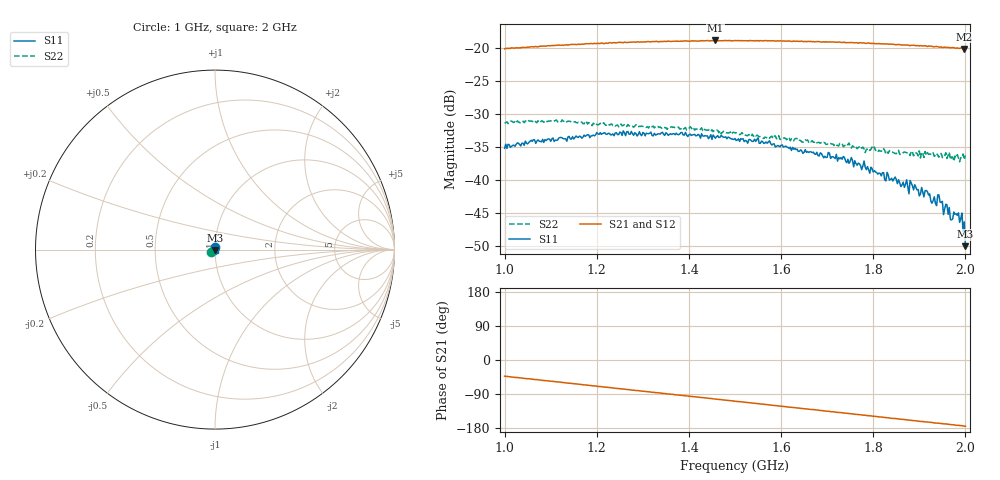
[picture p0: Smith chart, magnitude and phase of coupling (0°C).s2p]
!Agilent Technologies,E8363C,MY43030407,A.09.42.15
!Agilent E8363C: A.09.42.15
!Date: Friday, September 05, 2025 17:32:45
!Correction: S11(Full 2 Port(1,2))
!S21(Full 2 Port(1,2))
!S12(Full 2 Port(1,2))
!S22(Full 2 Port(1,2))
!S2P File: Measurements: S11, S21, S12, S22:
# Hz S  dB  R 50
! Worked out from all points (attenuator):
!   401 points, 1 GHz to 2 GHz, reference 50 ohm
!   highest |S21| = -18.78 dB at 1.458 GHz (marker M1); lowest = -20.1 dB at 1.998 GHz (marker M2)
!   lowest |S11| = -50.1 dB at 2 GHz (marker M3), VSWR 1.01, Z = 49.9 - j0.296 ohm
!   |S11| at or under -10 dB: start of sweep to end of sweep
!   |S22| runs from -37.2 to -30.9 dB; largest |S21 - S12| = 0.0015
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1e9  -35.19 98.9  -20.06 -42.7  -20.03 -42.7  -31.37 -145.9
1.06e9  -34.14 88.2  -19.73 -50.6  -19.74 -50.6  -31.07 -149.8
1.1675e9  -33.66 71.3  -19.34 -64.7  -19.37 -64.9  -31.22 -151.0
1.335e9  -32.98 41.4  -18.99 -86.9  -18.95 -86.9  -32.02 -157.6
1.4575e9  -33.66 18.7  -18.78 -103.1  -18.84 -103.1  -32.53 -157.1
1.5e9  -33.70 12.1  -18.80 -108.8  -18.81 -108.5  -32.85 -157.2
1.545e9  -34.14 -0.2  -18.81 -114.5  -18.83 -114.4  -33.33 -158.1
1.6675e9  -35.86 -26.9  -18.98 -130.8  -18.94 -130.9  -34.03 -157.4
1.75e9  -37.17 -46.5  -19.11 -141.6  -19.12 -141.7  -34.89 -153.4
1.835e9  -40.03 -61.0  -19.36 -152.8  -19.38 -152.9  -35.57 -149.1
1.8725e9  -39.99 -76.6  -19.49 -157.7  -19.48 -158.2  -35.85 -147.9
1.885e9  -40.90 -77.3  -19.51 -159.7  -19.53 -159.1  -35.67 -145.9
1.905e9  -41.15 -84.5  -19.61 -162.4  -19.57 -162.2  -35.81 -144.6
1.9175e9  -41.76 -85.0  -19.72 -163.8  -19.67 -163.5  -35.83 -143.9
1.9325e9  -42.56 -84.5  -19.74 -165.9  -19.70 -165.6  -36.42 -143.7
1.945e9  -43.37 -92.6  -19.81 -167.3  -19.75 -167.4  -36.04 -142.9
1.95e9  -43.27 -82.4  -19.87 -167.8  -19.77 -168.1  -36.58 -142.5
1.96e9  -43.80 -89.9  -19.85 -169.3  -19.84 -169.3  -36.74 -137.9
1.9675e9  -46.04 -94.3  -19.92 -170.5  -19.82 -170.4  -36.90 -139.2
1.9875e9  -46.47 -103.3  -19.97 -172.9  -19.99 -173.0  -37.23 -138.4
1.9975e9  -46.39 -114.5  -20.07 -174.5  -20.05 -174.4  -36.90 -139.7
2e9  -50.09 -108.8  -19.96 -174.7  -20.05 -174.9  -36.30 -137.5
